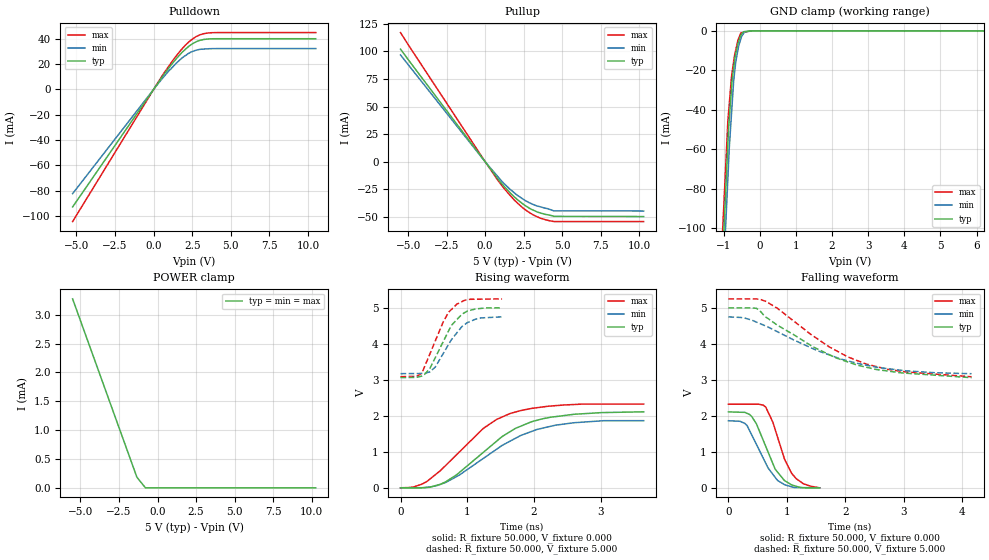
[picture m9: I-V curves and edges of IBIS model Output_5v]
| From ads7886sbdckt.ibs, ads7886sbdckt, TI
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[Model] Output_5v
Model_type 3-state
Vref=0.00000V
Rref=5.00000Mohms
Cref=50.0000pF
Vmeas=2.50000V
C_comp 1.513pF 1.513pF 1.513pF
| variable typ   min   max
[Voltage Range] 5.00000V 4.75000V 5.25000V
[POWER Clamp Reference] 5.00000V 4.75000V 5.25000V
[Pullup Reference] 5.00000V 4.75000V 5.25000V
[Pulldown Reference] 0.00000V 0.00000V 0.00000V
[GND Clamp Reference] 0.00000V 0.00000V 0.00000V
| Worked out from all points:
|   slope of the pulldown table from 0 to 0.75 V, typ, clamps not added: 57.3 ohm
|   slope of the pullup table from 0 to 0.75 V, typ, clamps not added: 54 ohm
|   GND clamp passes 1 mA (typ) near -0.47 V on its own axis
|   rising waveform, R_fixture 50.000, V_fixture 0.000: 20-80 % time 890ps typ, 960ps min, 818ps max; typ from 0.001 V to 2.11 V
|   falling waveform, R_fixture 50.000, V_fixture 0.000: 20-80 % time 346ps typ, 370ps min, 313ps max; typ from 2.11 V to 0.001 V
|   falling waveform, R_fixture 50.000, V_fixture 5.000: 20-80 % time 1.38ns typ, 1.42ns min, 1.26ns max; typ from 5 V to 3.06 V
|   rising waveform, R_fixture 50.000, V_fixture 5.000: 20-80 % time 337ps typ, 337ps min, 307ps max; typ from 3.06 V to 5 V
[GND Clamp]
-5.25V    -1.806A    -1.81A     -1.72A
-4.75V    -1.606A    -1.612A    -1.529A
-880mV    -57.6mA    -75.09mA   -45.85mA
-860mV    -49.59mA   -67.15mA   -41.38mA
-840mV    -44.6mA    -59.21mA   -36.91mA
-760mV    -24.61mA   -36.85mA   -20.86mA
-720mV    -18.95mA   -25.67mA   -15.55mA
-660mV    -11.58mA   -15.66mA   -9.611mA
-580mV    -5.38mA    -7.648mA   -3.784mA
-520mV    -2.156mA   -4.042mA   -1.089mA
-440mV    -442.5uA   -1.171mA   -754.2uA
10.5V     0A         0A         0A
[Pulldown]
-5.25V    -92.71mA   -82.21mA   -104.2mA
640mV     11.24mA    9.688mA    12.29mA
1.34V     22.25mA    18.96mA    24.41mA
1.76V     28.07mA    23.84mA    30.81mA
2.24V     33.48mA    28.16mA    36.91mA
2.52V     35.9mA     29.84mA    39.69mA
3V        38.58mA    31.45mA    42.94mA
3.74V     39.78mA    32.04mA    44.6mA
10.5V     39.87mA    32.09mA    44.71mA
[Pullup]
-5.5V     102mA      96.7mA     117mA
0V        -13.6uA    -14.3uA    32.8uA
760mV     -14.1mA    -12.4mA    -15.6mA
1.15V     -21mA      -18.7mA    -22.7mA
1.68V     -29mA      -25.6mA    -31.4mA
1.92V     -32.2mA    -28.5mA    -35.1mA
2.55V     -39.2mA    -34.7mA    -42.9mA
3V        -43.1mA    -38mA      -47.1mA
3.54V     -46.2mA    -40.7mA    -50.9mA
4.46V     -49.5mA    -44.5mA    -54.2mA
10.3V     -49.7mA    -44.7mA    -54.2mA
[POWER Clamp]
-5.5V     3.273mA    3.273mA    3.273mA
-5V       2.902mA    2.902mA    2.902mA
-4.5V     2.531mA    2.531mA    2.531mA
-1.337V   185.5uA    185.5uA    185.5uA
-780mV    0A         0A         0A
-390mV    0A         0A         0A
-250mV    0A         0A         0A
0V        0A         0A         0A
250mV     0A         0A         0A
9.75V     0A         0A         0A
10V       0A         0A         0A
10.25V    0A         0A         0A
[Rising Waveform]
R_fixture = 50.000
V_fixture = 0.000
V_fixture_min = 0.000
V_fixture_max = 0.000
|  time   V(typ)   V(min)   V(max)
0s        914.7uV    292.8uV    781.3uV
320ps     -1.45mV    1.997mV    100.4mV
680ps     171mV      151.7mV    628.2mV
1.24ns    985.5mV    816.7mV    1.652V
1.44ns    1.298V     1.074V     1.901V
1.64ns    1.56V      1.296V     2.064V
1.96ns    1.835V     1.564V     2.205V
2.32ns    1.977V     1.74V      2.282V
3.04ns    2.09V      1.865V     2.325V
3.64ns    2.111V     1.865V     2.325V
[Falling Waveform]
R_fixture = 50.000
V_fixture = 0.000
V_fixture_min = 0.000
V_fixture_max = 0.000
|  time   V(typ)   V(min)   V(max)
0s        2.111V     1.865V     2.325V
280ps     2.098V     1.791V     2.325V
360ps     2.042V     1.597V     2.325V
480ps     1.775V     1.203V     2.325V
640ps     1.145V     678.8mV    2.24V
800ps     516.6mV    291.8mV    1.618V
960ps     200.5mV    87.05mV    795.2mV
1.08ns    84.33mV    29.39mV    407.1mV
1.28ns    914.7uV    6.58mV     115.5mV
1.56ns    914.7uV    292.8uV    781.3uV
[Falling Waveform]
R_fixture = 50.000
V_fixture = 5.000
V_fixture_min = 4.750
V_fixture_max = 5.250
|  time   V(typ)   V(min)   V(max)
0s        5V         4.75V      5.249V
280ps     4.999V     4.717V     5.25V
480ps     4.988V     4.605V     5.251V
640ps     4.743V     4.495V     5.181V
840ps     4.516V     4.336V     4.986V
1.44ns    3.925V     3.872V     4.231V
2.04ns    3.5V       3.53V      3.64V
2.36ns    3.351V     3.409V     3.439V
3.04ns    3.185V     3.252V     3.221V
4.16ns    3.061V     3.171V     3.087V
[Rising Waveform]
R_fixture = 50.000
V_fixture = 5.000
V_fixture_min = 4.750
V_fixture_max = 5.250
|  time   V(typ)   V(min)   V(max)
0s        3.061V     3.171V     3.087V
240ps     3.068V     3.175V     3.097V
320ps     3.105V     3.177V     3.186V
440ps     3.318V     3.221V     3.721V
520ps     3.616V     3.354V     4.079V
720ps     4.361V     3.985V     4.877V
840ps     4.667V     4.297V     5.099V
920ps     4.823V     4.482V     5.173V
1.12ns    4.968V     4.683V     5.239V
1.52ns    5V         4.75V      5.249V
[Ramp]
| variable typ min max
dV/dt_r 1.26648/786.328p 1.11824/845.297p 1.39500/720.124p
dV/dt_f 1.16336/1.27979n 947.628m/1.41381n 1.29743/1.18640n
R_load = 50.0000Ohms
